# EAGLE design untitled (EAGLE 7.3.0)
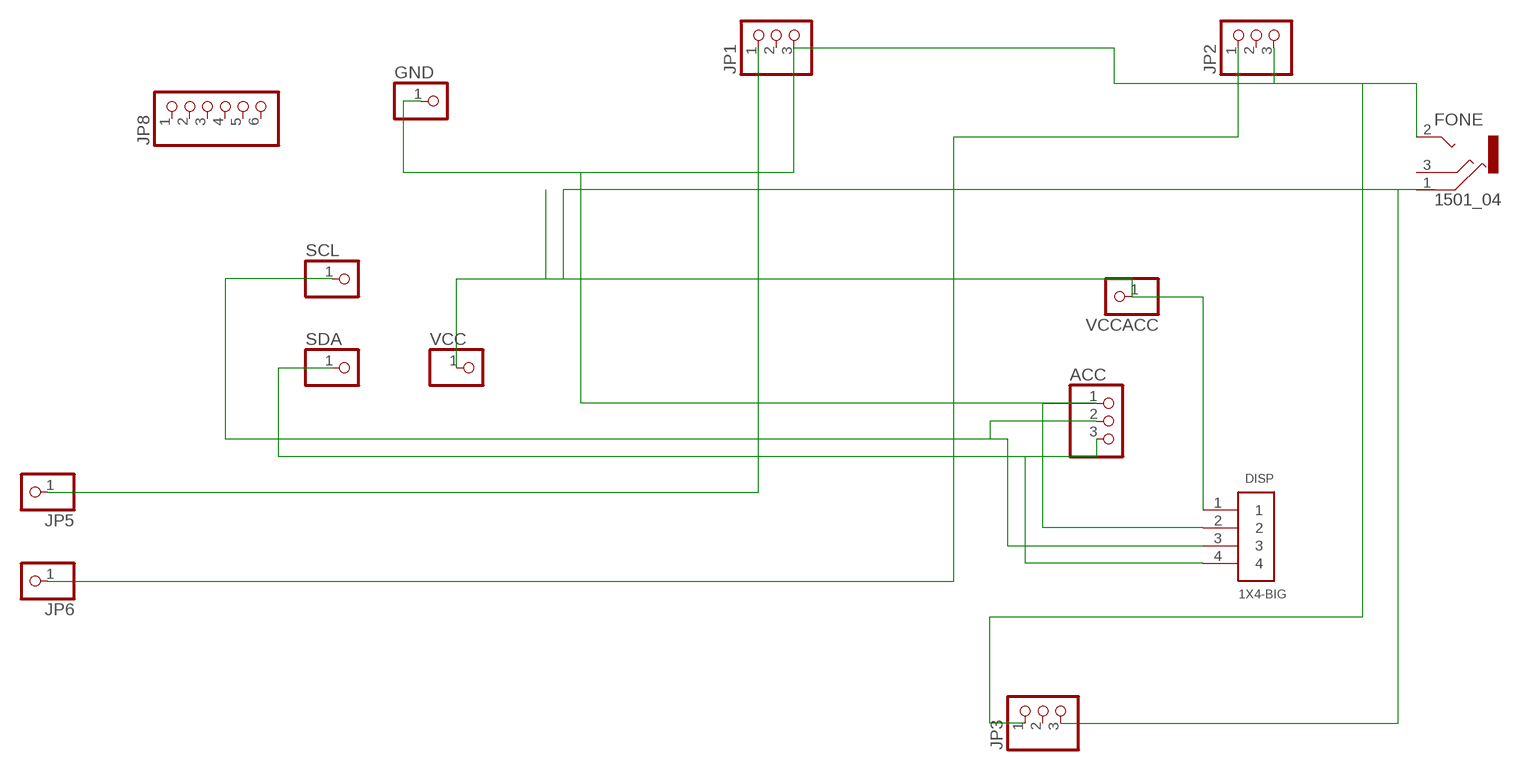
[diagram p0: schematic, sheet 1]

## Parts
ACC  PINHD-1X3  [1X03]
DISP  1X4-BIG  [1X04-BIG]
FONE  1501_04  [1501_05]
GND  PINHD-1X1  [1X01]
JP1  PINHD-1X3  [1X03]
JP2  PINHD-1X3  [1X03]
JP3  PINHD-1X3  [1X03]
JP5  PINHD-1X1  [1X01]
JP6  PINHD-1X1  [1X01]
JP8  PINHD-1X6  [1X06]
SCL  PINHD-1X1  [1X01]
SDA  PINHD-1X1  [1X01]
VCC  PINHD-1X1  [1X01]
VCCACC  PINHD-1X1  [1X01]

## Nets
N$1: ACC.2 DISP.3 SCL.1
N$2: ACC.3 DISP.4 SDA.1
N$3: ACC.1 DISP.2 FONE.2 GND.1 JP1.3 JP2.3 JP3.1
N$4: DISP.1 FONE.1 JP3.3 VCC.1 VCCACC.1
N$5: JP1.1 JP5.1
N$6: JP2.1 JP6.1
Unconnected: FONE.3 JP1.2 JP2.2 JP3.2 JP8.1 JP8.2 JP8.3 JP8.4 JP8.5 JP8.6

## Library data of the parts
ACC JP1-JP3 = adafruit:PINHD-1X3: PIN HEADER
DISP = adafruit:1X4: 4-pin connector
FONE = con-lumberg:1501_0*: Jack connectors according to JISC 6560, 2.5 mm Klinkensteckverbinder nach JISC 6560, 2,5 mm Source: http://www.lumberg.com/Produkte/PDFs/1501_05.pdfedit 1501_03 http://www.lumberg.com/Produkte/PDFs/1501_06.pdf; OC_FARNELL: 1216977; OC_NEWARK: unknown
GND JP5 JP6 SCL SDA VCC VCCACC = adafruit:PINHD-1X1: Pin header 1x1 for 0.1" spacing
JP8 = adafruit:PINHD-1X6: PIN HEADER

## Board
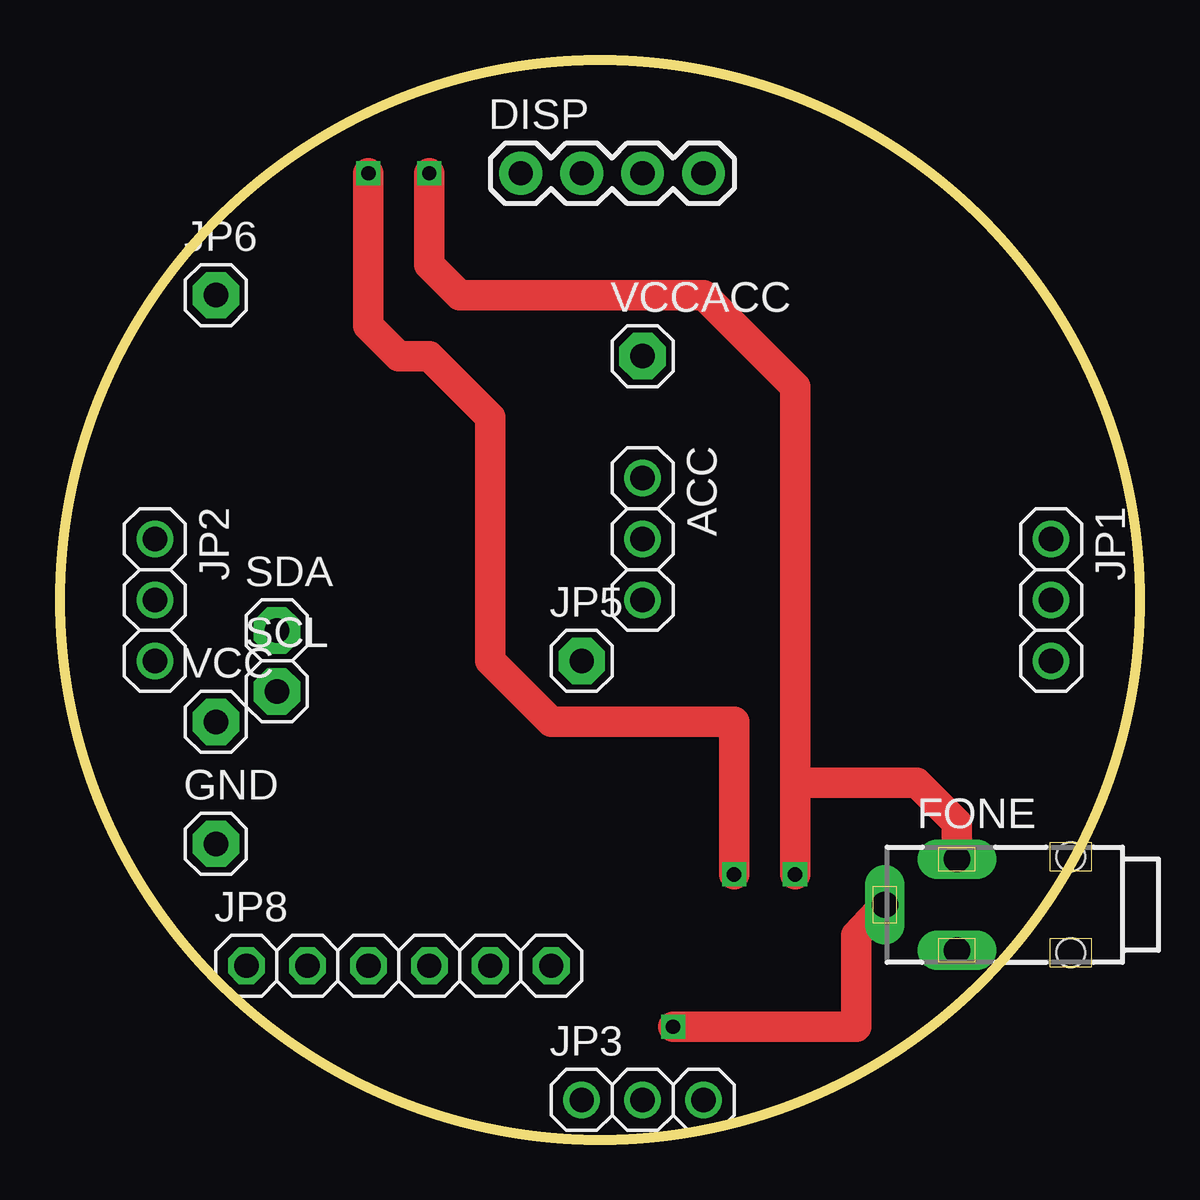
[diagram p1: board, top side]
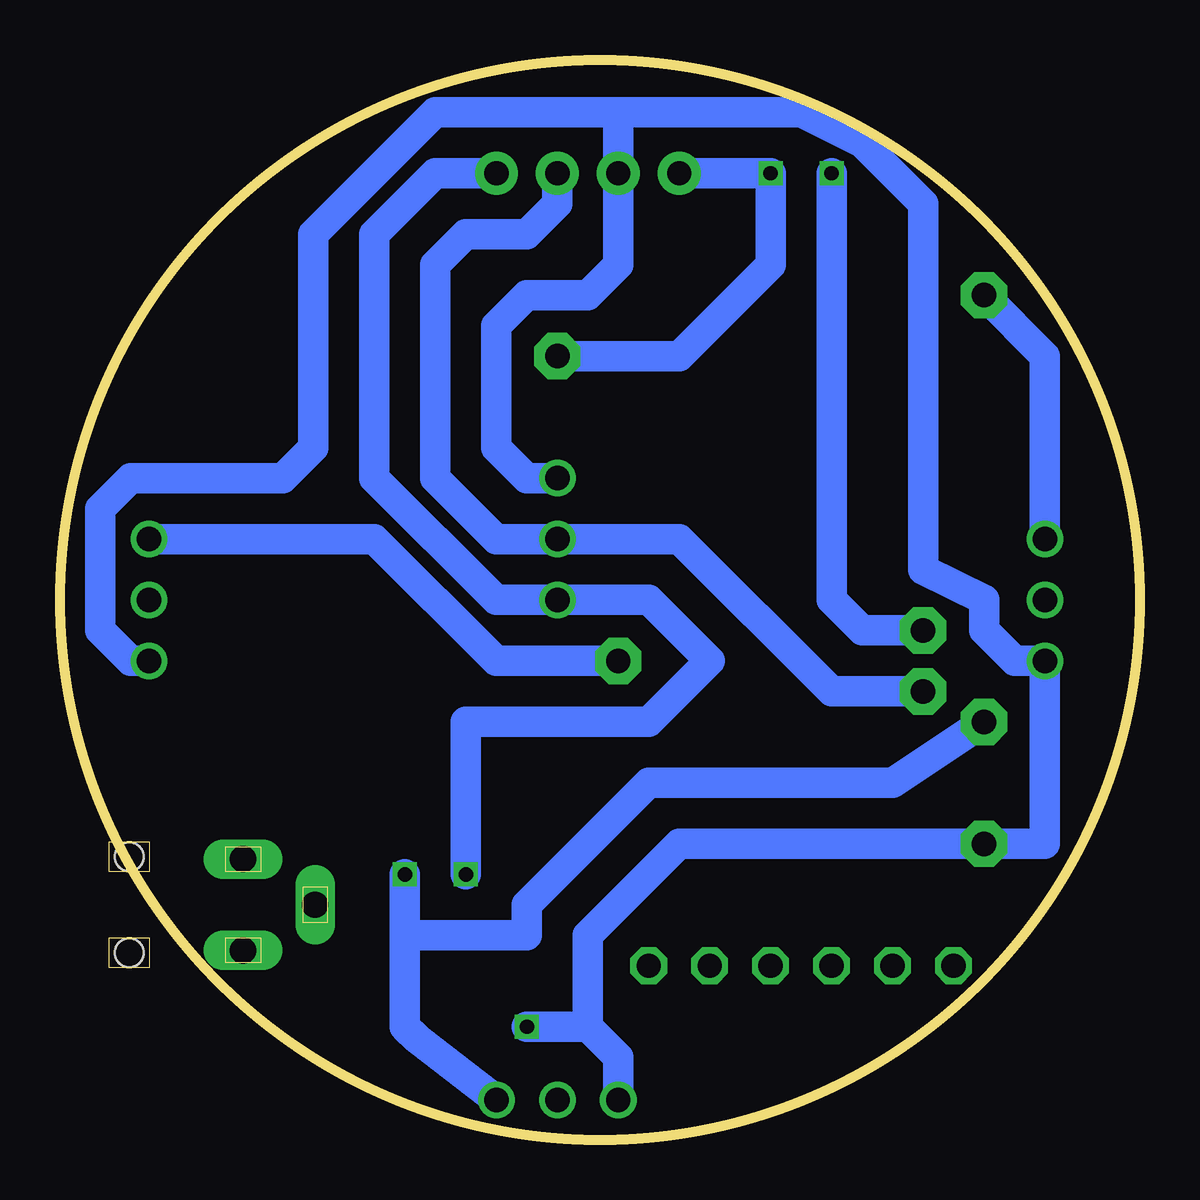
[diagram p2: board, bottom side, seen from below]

Size 45 x 45 mm. Coordinates in mm from the lower left corner, seen from the top.
Outline: circle at 22.5,22.5 radius 22.5
Copper layers (1*16): Top 0.035mm / dielectric 1.5mm / Bottom 0.035mm
Design rules "default": minimum track width 10mil, minimum drill 24mil, track to track 8mil, track to pad 8mil, pad to pad 8mil, via to via 8mil, smd to smd 8mil, copper to edge 40mil, drill to drill 8mil, minimum pad ring 10mil, minimum via ring 8mil, stop-mask expansion 4mil, vias tented up to drill 0mil, thermal gap 10mil

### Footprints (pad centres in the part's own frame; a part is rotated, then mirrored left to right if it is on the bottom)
1X03 = drill 1.016: 1 -2.54,0; 2 0,0; 3 2.54,0
1X04-BIG = drill 1.016 pad 1.778: 1 0,0; 2 2.54,0; 3 5.08,0; 4 7.62,0
1501_05 = drill 1.1 pad 1.4 long: 1 -1.9,-8.5; 2 0,-11.5; 3 1.9,-8.5 | hole 1.2: -2,-3.75; 2,-3.75
1X01 = drill 1.016 pad 1.93 octagon: 1 0,0
1X06 = drill 1.016 octagon: 1 -6.35,0; 2 -3.81,0; 3 -1.27,0; 4 1.27,0; 5 3.81,0; 6 6.35,0

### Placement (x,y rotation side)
ACC  24.28,25.04 270 top
DISP  19.2,40.28 0 top
FONE  45.87,9.8 270 top
GND  6.5,12.34 0 top
JP1  41.3,22.5 270 top
JP2  3.96,22.5 270 top
JP3  24.28,1.67 0 top
JP5  21.74,19.96 0 top
JP6  6.5,35.2 0 top
JP8  14.12,7.26 0 top
SCL  9.04,18.69 0 top
SDA  9.04,21.23 0 top
VCC  6.5,17.42 0 top
VCCACC  24.28,32.66 0 top

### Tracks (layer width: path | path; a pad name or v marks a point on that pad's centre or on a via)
N$1
  Bottom 1.27: SCL.1 12.85,18.69 19.2,25.04 ACC.2 26.82,25.04 29.36,27.58 29.36,36.47 28.09,37.74 25.55,37.74 24.28,39.01 DISP.3
N$2  (via drill 0.6)
  Top 1.27: v28.09,11.07 28.09,17.42 20.47,17.42 17.93,19.96 17.93,30.12 15.39,32.66 14.12,32.66 12.85,33.93 v12.85,40.28
  Bottom 1.27: DISP.4 29.36,40.28 31.9,37.74 31.9,27.58 26.82,22.5 ACC.3 20.47,22.5 17.93,19.96 20.47,17.42 28.09,17.42 v28.09,11.07 | v12.85,40.28 12.85,22.5 11.58,21.23 SDA.1
N$3  (via drill 0.6)
  Top 1.27: FONE.2 33.17,8.53 33.17,4.72 v25.55,4.72
  Bottom 1.27: JP1.3 42.06,19.96 43.33,21.23 43.33,26.31 42.06,27.58 35.71,27.58 34.44,28.85 34.44,37.74 29.36,42.82 21.74,42.82 | 21.74,42.82 14.12,42.82 11.58,41.55 9.04,39.01 9.04,23.77 6.5,22.5 6.5,21.23 5.23,19.96 JP2.3 3.96,12.34 GND.1 19.2,12.34 23.01,8.53 23.01,4.72 | ACC.1 25.55,27.58 26.82,28.85 26.82,33.93 25.55,35.2 23.01,35.2 21.74,36.47 DISP.2 21.74,42.82 | JP3.1 21.74,3.45 23.01,4.72 | v25.55,4.72 23.01,4.72
N$4  (via drill 0.6)
  Top 1.27: v15.39,40.28 15.39,36.47 16.66,35.2 26.82,35.2 30.63,31.39 30.63,14.88 | 30.63,14.88 v30.63,11.07 | FONE.1 37.37,13.22 35.71,14.88 30.63,14.88
  Bottom 1.27: DISP.1 v15.39,40.28 15.39,36.47 19.2,32.66 VCCACC.1 | VCC.1 10.31,14.88 20.47,14.88 25.55,9.8 25.55,8.53 30.63,8.53 | 30.63,8.53 v30.63,11.07 | JP3.3 30.12,4.21 30.63,4.72 30.63,8.53
N$5
  Bottom 1.27: JP1.1 31.9,25.04 26.82,19.96 JP5.1
N$6
  Bottom 1.27: JP2.1 3.96,32.66 JP6.1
